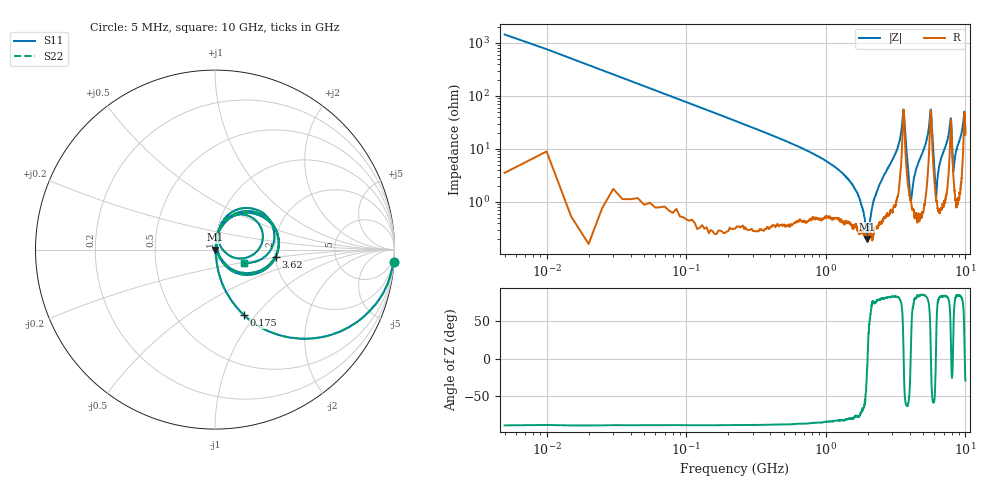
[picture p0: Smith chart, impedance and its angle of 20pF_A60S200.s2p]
! Amotech Co.,Ltd.
! http://www.amotech.co.kr/
! Part Number: A60S200
! These Parameters are Measured in Series Mode Connection
! Operation Temp=25[degC], DC Bias Voltage=0[V]
! Freq. Start=5[MHz] Stop=10[GHz], 2000[Steps]
! Date: Monday, July 13, 2020, 01:38:02
# GHZ S RI R 50.000000
!Freq.(Hz) S11(Real) S11(Imag) S21(Real) S21(Imag) S12(Real) S12(Imag) S22(Real) S22(Imag)
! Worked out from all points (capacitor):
!   2000 points, 5 MHz to 10 GHz, reference 50 ohm
!   read as one part in series: C = 20.8 pF near 55 MHz
!   lowest |Z| = 200 mohm at 1.975 GHz (marker M1)
!   series resonance near 1.991 GHz, so ESL is about 310 pH
!   S11 on the Smith chart (normalised r, x): 5 MHz: 1, -29; 175 MHz: 1.01, -0.87; 3.62 GHz: 2.02, -0.18; 10 GHz: 1.37, -0.21
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0.005  0.995 -0.0691  0.00497 0.0691  0.00497 0.0691  0.995 -0.0691
0.075  0.5098 -0.4965  0.4902 0.4965  0.4902 0.4965  0.5098 -0.4965
0.175  0.1618 -0.365  0.8382 0.365  0.8382 0.365  0.1618 -0.365
0.58  0.0187 -0.1209  0.9813 0.1209  0.9813 0.1209  0.0187 -0.1209
1.675  0.00363 -0.0146  0.9964 0.0146  0.9964 0.0146  0.00363 -0.0146
1.975  0.00196 -0.000422  0.998 0.000422  0.998 0.000422  0.00196 -0.000422
2.385  0.00398 0.0185  0.996 -0.0185  0.996 -0.0185  0.00398 0.0185
3.34  0.0316 0.1183  0.9684 -0.1183  0.9684 -0.1183  0.0316 0.1183
3.53  0.1748 0.2042  0.8252 -0.2042  0.8252 -0.2042  0.1748 0.2042
3.62  0.3406 -0.0386  0.6594 0.0386  0.6594 0.0386  0.3406 -0.0386
4.065  0.0103 0.00121  0.9897 -0.00121  0.9897 -0.00121  0.0103 0.00121
4.435  0.00785 0.0407  0.9921 -0.0407  0.9921 -0.0407  0.00785 0.0407
5.005  0.0152 0.0925  0.9848 -0.0925  0.9848 -0.0925  0.0152 0.0925
5.53  0.1737 0.2148  0.8263 -0.2148  0.8263 -0.2148  0.1737 0.2148
5.66  0.3527 0.0092  0.6473 -0.0092  0.6473 -0.0092  0.3527 0.0092
6.165  0.011 0.00374  0.989 -0.00374  0.989 -0.00374  0.011 0.00374
6.67  0.0114 0.0618  0.9886 -0.0618  0.9886 -0.0618  0.0114 0.0618
7.84  0.2506 0.1328  0.7494 -0.1328  0.7494 -0.1328  0.2506 0.1328
8.16  0.0371 0.00811  0.9629 -0.00811  0.9629 -0.00811  0.0371 0.00811
8.335  0.0198 0.0508  0.9802 -0.0508  0.9802 -0.0508  0.0198 0.0508
9.78  0.2853 0.1871  0.7147 -0.1871  0.7147 -0.1871  0.2853 0.1871
10  0.1624 -0.0742  0.8376 0.0742  0.8376 0.0742  0.1624 -0.0742
